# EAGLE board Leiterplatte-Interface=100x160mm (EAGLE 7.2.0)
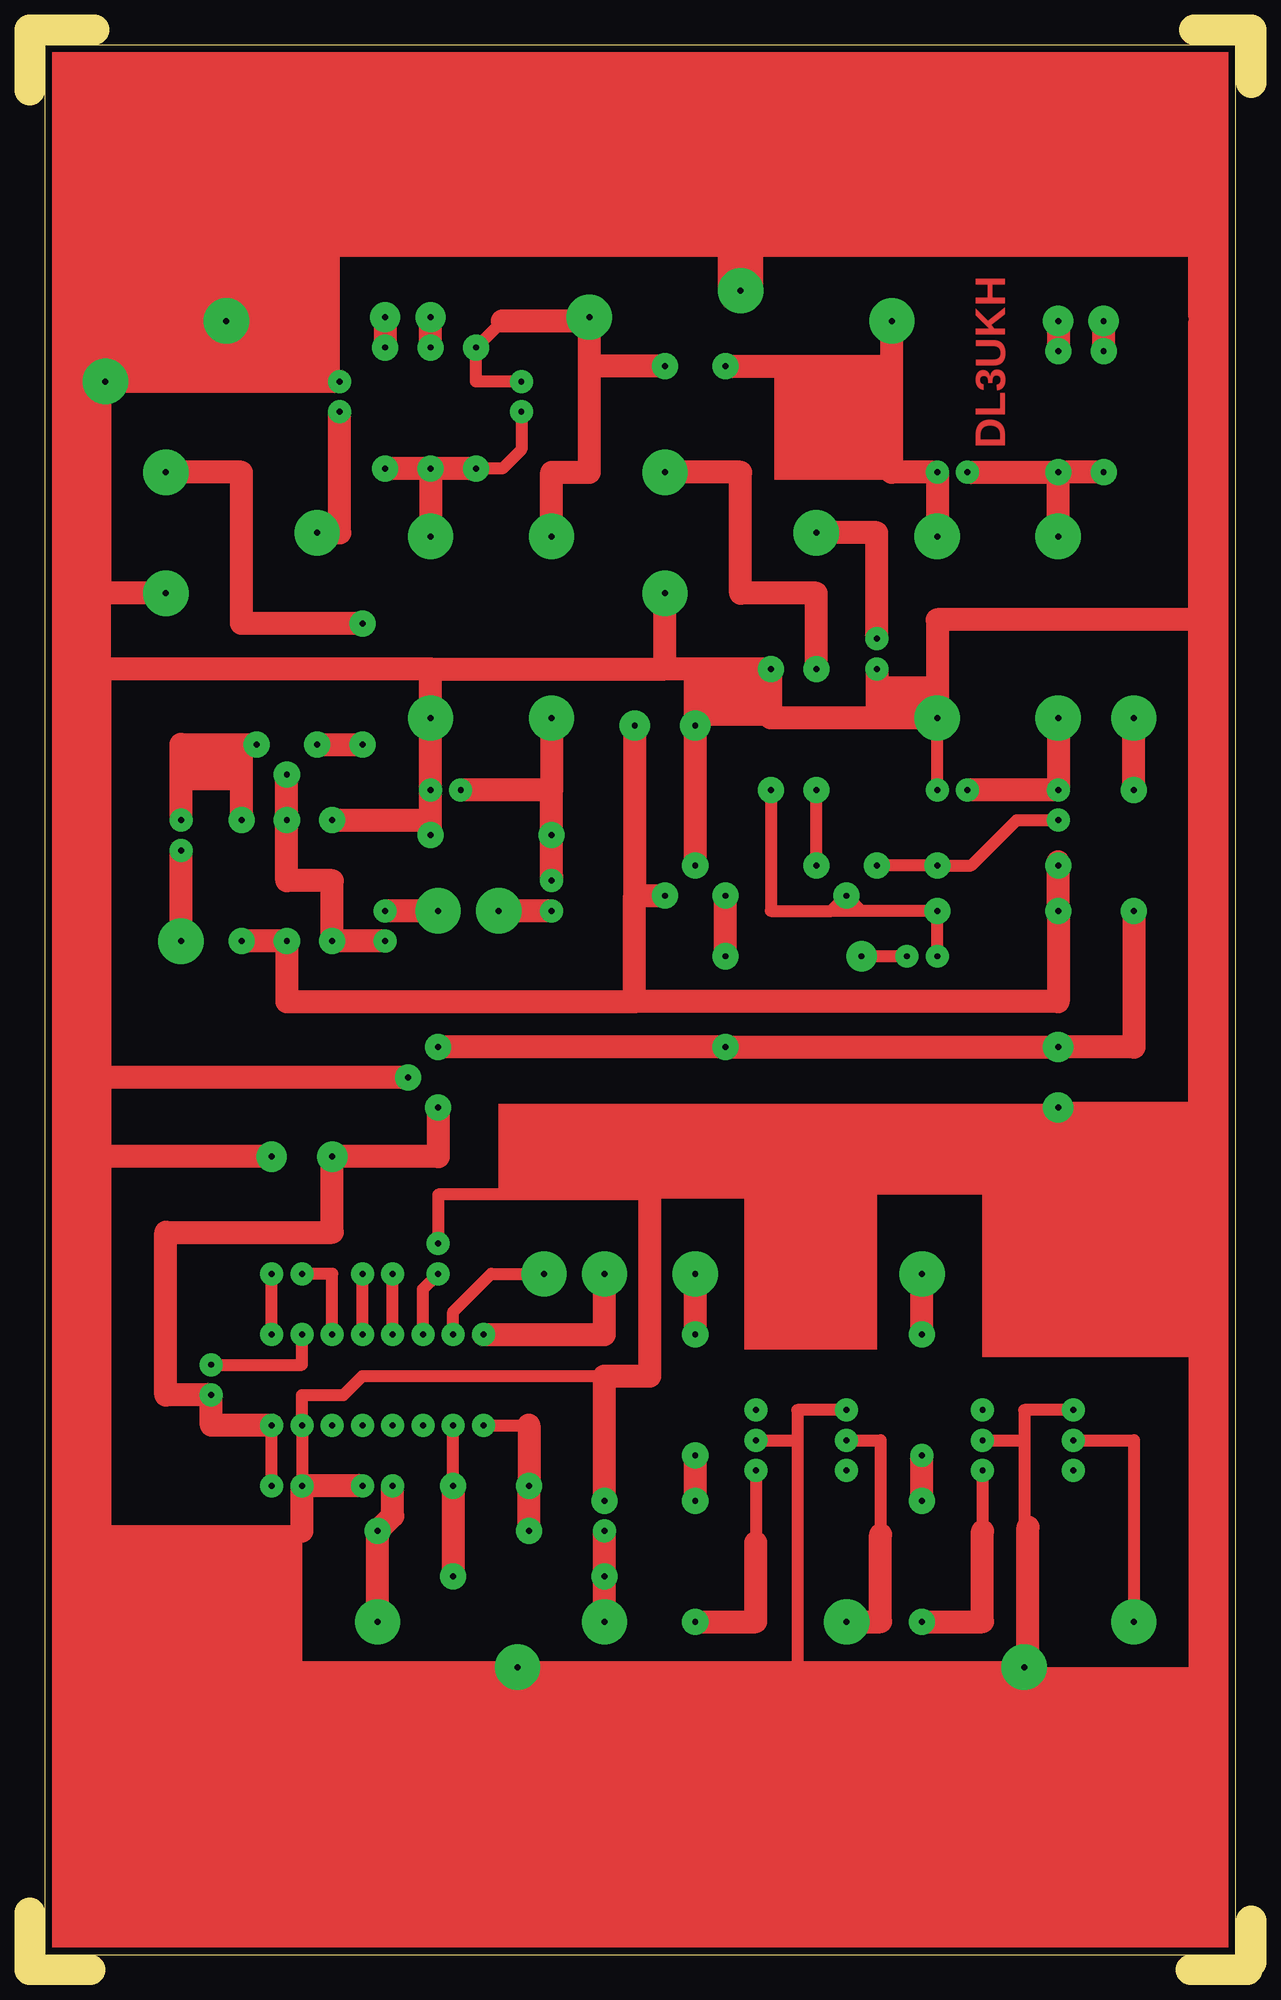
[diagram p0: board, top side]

Size 102.55 x 162.88 mm. Coordinates in mm from the lower left corner, seen from the top.
Outline: 5.4,162.88 0.32,162.88
Outline: 0,162.88 0,157.8
Outline: 97.79,162.88 102.55,162.88 102.55,158.43
Outline: 5.08,0 0,0 0,4.76
Outline: 102.55,4.13 102.55,0.64
Outline: 97.47,0 102.23,0
Outline: 1.27,161.61 101.28,161.61 101.28,1.27 1.27,1.27 1.27,161.61
Copper layers (1*16): Top 0.035mm / dielectric 1.5mm / Bottom 0.035mm
Design rules "default": minimum track width 10mil, minimum drill 24mil, track to track 8mil, track to pad 8mil, pad to pad 8mil, via to via 8mil, smd to smd 8mil, copper to edge 40mil, drill to drill 8mil, minimum pad ring 10mil, minimum via ring 8mil, stop-mask expansion 4mil, vias tented up to drill 0mil, thermal gap 10mil

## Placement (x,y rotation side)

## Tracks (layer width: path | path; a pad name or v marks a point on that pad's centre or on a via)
S$1  (via drill 0.5 pad 1.93, 0.5 pad 2.18)
  Top 1.016: 69.85,88.9 v76.2,88.9 v76.2,85.09 | 69.85,88.9 v68.58,90.17 67.31,88.9 | 67.31,88.9 62.23,88.9 v62.23,99.06 | 69.85,88.9 67.31,88.9
S$2  (via drill 0.5 pad 3.81)
  other vias: 72.39,138.43
S$3  (via drill 0.5 pad 2.18, 0.5 pad 2.54)
  Top 1.93: v86.36,138.43 v86.36,135.89
S$4  (via drill 0.5 pad 1.93, 0.5 pad 2.54)
  Top 1.016: v73.66,85.09 v69.85,85.09
S$5  (via drill 0.5 pad 2.18, 0.5 pad 2.54)
  Top 1.93: v90.17,135.89 v90.17,138.43
S$6  (via drill 0.5 pad 2.18, 0.5 pad 2.54)
  Top 1.93: 86.36,93.03 v86.36,88.9 86.36,81.28 50.8,81.28 | v17.78,86.36 v21.59,86.36 21.59,81.28 50.8,81.28 | 50.8,81.28 50.8,90.17 | 50.8,90.17 v53.34,90.17 | v50.8,104.46 50.8,90.17
S$7
  Top 1.016: 97.79,138.75 97.79,145.42
S$8  (via drill 0.5 pad 1.93, 0.5 pad 3.81)
  Top 1.93: v86.36,105.09 v86.36,99.06 v78.74,99.06
S$9  (via drill 0.5 pad 1.93, 0.5 pad 3.81)
  Top 1.93: v24.13,120.65 26.04,120.65 v26.04,130.81
S$10  (via drill 0.5 pad 1.93, 0.5 pad 3.81)
  Top 1.93: v71.12,111.76 71.12,120.65 v66.04,120.65
S$11  (via drill 0.5 pad 1.93, 0.5 pad 2.18, 0.5 pad 3.81)
  Top 1.93: v43.82,105.09 43.82,99.06 | 43.82,99.06 v36.2,99.06 | 43.82,99.06 v43.82,95.25 43.82,91.76
S$12  (via drill 0.5 pad 1.93, 0.5 pad 2.18, 0.5 pad 3.81)
  Top 1.93: v90.17,125.73 v86.36,125.73 | v86.36,120.33 v86.36,125.73 | v78.74,125.73 v86.36,125.73
S$13  (via drill 0.5 pad 2.18)
  other vias: 86.36,92.71
S$14  (via drill 0.5 pad 2.18)
  Top 1.93: v24.13,102.87 v27.94,102.87
S$15  (via drill 0.5 pad 3.81)
  Top 1.93: 33.66,125.73 v33.66,120.33
S$16  (via drill 0.5 pad 1.93)
  other vias: 43.82,91.44
S$17  (via drill 0.5 pad 2.18)
  Top 1.93: v31.75,74.93 6.67,74.93
S$18  (via drill 0.5 pad 1.93, 0.5 pad 2.18)
  Top 1.016: v71.12,92.71 v76.2,92.71 79.06,92.71 82.87,96.52 86.04,96.52 86.36,96.84 v86.36,96.52
S$19  (via drill 0.5 pad 2.18, 0.5 pad 2.54)
  Top 1.93: v29.84,138.75 v29.84,136.21
S$20  (via drill 0.5 pad 2.18, 0.5 pad 2.54)
  Top 1.93: v33.66,136.21 v33.66,138.75
S$21  (via drill 0.5 pad 2.18)
  Top 1.016: v66.04,92.71 v66.04,99.06
S$22  (via drill 0.5 pad 1.93, 0.5 pad 3.81)
  Top 1.93: v43.82,88.9 v39.37,88.9
S$23  (via drill 0.5 pad 2.18, 0.5 pad 3.81)
  Top 1.93: v66.04,109.22 66.04,115.57 59.69,115.57 59.69,125.73 v53.34,125.73
S$24  (via drill 0.5 pad 1.93, 0.5 pad 2.18)
  Top 1.016: v35.56,40.64 v35.56,45.72
  Top 1.93: v35.56,40.64 v35.56,33.02
S$25  (via drill 0.5 pad 1.93, 0.5 pad 2.18)
  Top 1.016: v41.28,130.81 41.28,127.63 39.69,126.05 v37.47,126.05
  Top 1.93: v29.84,126.05 v33.66,126.05 v37.47,126.05
S$26  (via drill 0.5 pad 1.93, 0.5 pad 3.81)
  Top 1.016: v35.56,53.34 35.56,55.25 38.74,58.42 v43.18,58.42
S$27  (via drill 0.5 pad 1.93, 0.5 pad 2.18, 0.5 pad 3.81)
  Top 1.016: v41.28,133.35 37.47,133.35 v37.47,136.21 39.69,138.43 | 46.99,139.06 46.99,138.43
  Top 1.93: v43.82,120.33 43.82,125.73 46.99,125.73 46.99,134.62 | 46.99,134.62 46.99,138.43 39.69,138.43 | v53.34,134.62 46.99,134.62
S$28  (via drill 0.5 pad 1.93, 0.5 pad 2.18, 0.5 pad 3.81)
  Top 1.93: v76.2,120.33 v76.2,125.73 72.39,125.73 72.39,134.62 | 72.39,134.62 72.39,138.75 | v58.42,134.62 72.39,134.62
S$29  (via drill 0.5 pad 3.81)
  other vias: 46.99,138.75
S$30  (via drill 0.5 pad 1.93, 0.5 pad 3.81)
  Top 1.93: v34.29,88.9 v29.84,88.9
S$31  (via drill 0.5 pad 2.18, 0.5 pad 3.81)
  Top 1.93: v27.94,113.03 17.78,113.03 17.78,125.73 v11.43,125.73
S$32  (via drill 0.5 pad 1.93, 0.5 pad 2.18)
  Top 1.93: v29.84,86.36 v25.4,86.36 25.4,91.44 21.59,91.44 v21.59,96.52 v21.59,100.33
S$33  (via drill 0.5 pad 2.18, 0.5 pad 2.54)
  Top 1.93: v34.29,77.47 v58.42,77.47 v86.36,77.47 92.71,77.47 v92.71,88.9
S$34  (via drill 0.5 pad 1.93, 0.5 pad 3.81)
  Top 1.93: v38.1,53.34 48.26,53.34 v48.26,58.42
S$35  (via drill 0.5 pad 2.18, 0.5 pad 3.81)
  Top 1.016: 92.71,99.38 v92.71,99.06
  Top 1.93: v92.71,99.06 v92.71,105.09
S$36  (via drill 0.5 pad 2.18)
  Top 1.93: v58.42,85.09 v58.42,90.17
S$37  (via drill 0.5 pad 1.93)
  other vias: 20.32,58.42
S$38  (via drill 0.5 pad 1.93)
  Top 1.016: v15.24,50.8 22.86,50.8 v22.86,53.34
S$39  (via drill 0.5 pad 1.93, 0.5 pad 2.18, 0.5 pad 2.54)
  Top 1.016: 33.97,72.39 v34.29,72.39 | v20.32,40.64 v20.32,45.72
  Top 1.93: v20.32,45.72 15.24,45.72 v15.24,48.26 11.43,48.26 11.43,61.91 25.4,61.91 v25.4,68.26 34.29,68.26 v34.29,72.39
S$40  (via drill 0.5 pad 1.93)
  Top 1.016: v33.02,53.34 33.02,57.15 v34.29,58.42
S$41  (via drill 0.5 pad 1.93)
  Top 1.016: v30.48,53.34 v30.48,58.42
S$42  (via drill 0.5 pad 1.93)
  Top 1.016: v27.94,53.34 27.94,58.74
S$43  (via drill 0.5 pad 1.93)
  Top 1.016: v25.4,53.34 25.4,58.42 v22.86,58.42
S$44  (via drill 0.5 pad 1.93)
  other vias: 80.01,46.99
S$45  (via drill 0.5 pad 1.93)
  Top 1.016: v20.32,53.34 20.32,58.74
S$46  (via drill 0.5 pad 1.93, 0.5 pad 2.18)
  Top 1.016: v80.01,41.91 80.01,36.83
  Top 1.93: v74.93,29.21 80.01,29.21 80.01,36.83
S$47  (via drill 0.5 pad 1.93)
  other vias: 87.63,41.91
S$48  (via drill 0.5 pad 1.93)
  other vias: 33.02,45.72
S$49  (via drill 0.5 pad 1.93)
  other vias: 30.48,45.72
S$50  (via drill 0.5 pad 1.93)
  other vias: 27.94,45.72
S$51  (via drill 0.5 pad 1.93)
  other vias: 25.4,45.72
S$52  (via drill 0.5 pad 1.93, 0.5 pad 2.18)
  Top 1.016: v38.1,45.72 41.91,45.72
  Top 1.93: 41.91,45.72 v41.91,40.64 v41.91,36.83
S$53  (via drill 0.5 pad 1.93)
  other vias: 27.94,58.42
S$54  (via drill 0.5 pad 1.93, 0.5 pad 3.81)
  Top 1.016: v87.63,44.45 92.71,44.45 v92.71,29.21
S$55  (via drill 0.5 pad 3.81)
  other vias: 16.51,138.43
S$56  (via drill 0.5 pad 1.93, 0.5 pad 2.18)
  Top 1.93: v74.93,39.37 v74.93,43.18
S$57  (via drill 0.5 pad 1.93, 0.5 pad 2.18, 0.5 pad 3.81)
  Top 1.93: v30.48,40.64 30.48,38.1 v29.21,36.83 v29.21,29.21
S$58  (via drill 0.5 pad 2.18, 0.5 pad 3.81)
  Top 1.93: v74.93,53.34 v74.93,58.42
S$59  (via drill 0.5 pad 1.93)
  other vias: 60.96,46.99
S$60  (via drill 0.5 pad 1.93, 0.5 pad 2.18)
  Top 1.016: 17.78,101.6 v19.05,102.87
  Top 1.93: v17.78,96.52 17.78,101.6 | v12.7,96.52 12.7,102.87 v19.05,102.87
S$61  (via drill 0.5 pad 1.93, 0.5 pad 2.18)
  Top 1.016: v60.96,41.91 60.96,35.88
  Top 1.93: v55.88,29.21 60.96,29.21 60.96,35.88
S$62  (via drill 0.5 pad 1.93)
  other vias: 68.58,41.91
S$63  (via drill 0.5 pad 1.93, 0.5 pad 3.81)
  Top 1.016: v68.58,44.45 71.44,44.45 71.44,36.51 | 68.9,29.21 v68.58,29.21
  Top 1.93: 68.9,29.21 71.44,29.21 71.44,36.51
S$64
  Top 1.93: 83.82,25.4 83.82,37.15
S$65  (via drill 0.5 pad 2.18)
  Top 1.93: v55.88,39.37 v55.88,43.18
S$66  (via drill 0.5 pad 1.93, 0.5 pad 2.18, 0.5 pad 3.81)
  Top 1.93: v48.26,29.21 v48.26,33.02 v48.26,36.83
S$67  (via drill 0.5 pad 2.18, 0.5 pad 3.81)
  Top 1.93: v55.88,53.34 v55.88,58.42
S$68  (via drill 0.5 pad 1.93, 0.5 pad 3.81)
  Top 1.93: v12.7,86.36 v12.7,93.98
S$70  (via drill 0.5 pad 1.93, 0.5 pad 2.18, 0.5 pad 2.54, 0.5 pad 3.81)
  Top 1.016: v60.96,44.45 64.45,44.45 | 64.45,44.45 64.45,25.4 v40.96,25.4 | v40.96,25.4 6.35,25.4 6.35,36.83 | v86.36,72.39 97.79,72.39 | 97.79,72.39 97.79,113.35 97.79,138.43 | v76.2,99.06 v76.2,105.09 | v6.35,133.35 6.35,115.57 6.35,109.22 6.35,68.26 6.35,36.83 | 6.35,36.83 22.86,36.83 | v22.86,40.64 v22.86,45.72 22.86,48.26 26.35,48.26 27.94,49.85 48.26,49.85 | 52.07,65.09 34.29,65.09 v34.29,60.96 | v68.58,46.99 64.45,46.99 64.45,44.45 | v80.01,44.45 83.5,44.45 | 83.5,44.45 v83.5,25.4 v40.96,25.4 | v87.63,46.99 83.5,46.99 83.5,44.45 | 97.79,72.39 97.79,24.77
  Top 1.93: v33.66,95.25 33.66,96.52 | 33.66,96.52 v33.66,99.06 v33.66,105.09 33.66,109.22 | 71.12,105.09 v76.2,105.09 76.2,113.35 97.79,113.35 | 71.12,105.09 62.23,105.09 v62.23,109.22 55.88,109.22 | v71.12,109.22 71.12,105.09 | 55.88,109.22 53.34,109.22 | 53.34,109.22 v53.34,115.57 | 33.66,109.22 53.34,109.22 | v25.4,96.52 33.66,96.52 | 33.66,109.22 6.35,109.22 | v55.88,92.71 v55.88,104.46 55.88,109.22 | v26.04,133.35 v6.35,133.35 | v11.43,115.57 6.35,115.57 | 22.86,36.83 v22.86,40.64 v27.94,40.64 | v20.32,68.26 6.35,68.26 | 52.07,65.09 52.07,49.85 48.26,49.85 v48.26,39.37
  Top 3.81: v59.69,140.97 59.69,145.73
(copper drawn outside any net)
  shapes: Top area x18

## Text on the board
Top: DL3UKH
